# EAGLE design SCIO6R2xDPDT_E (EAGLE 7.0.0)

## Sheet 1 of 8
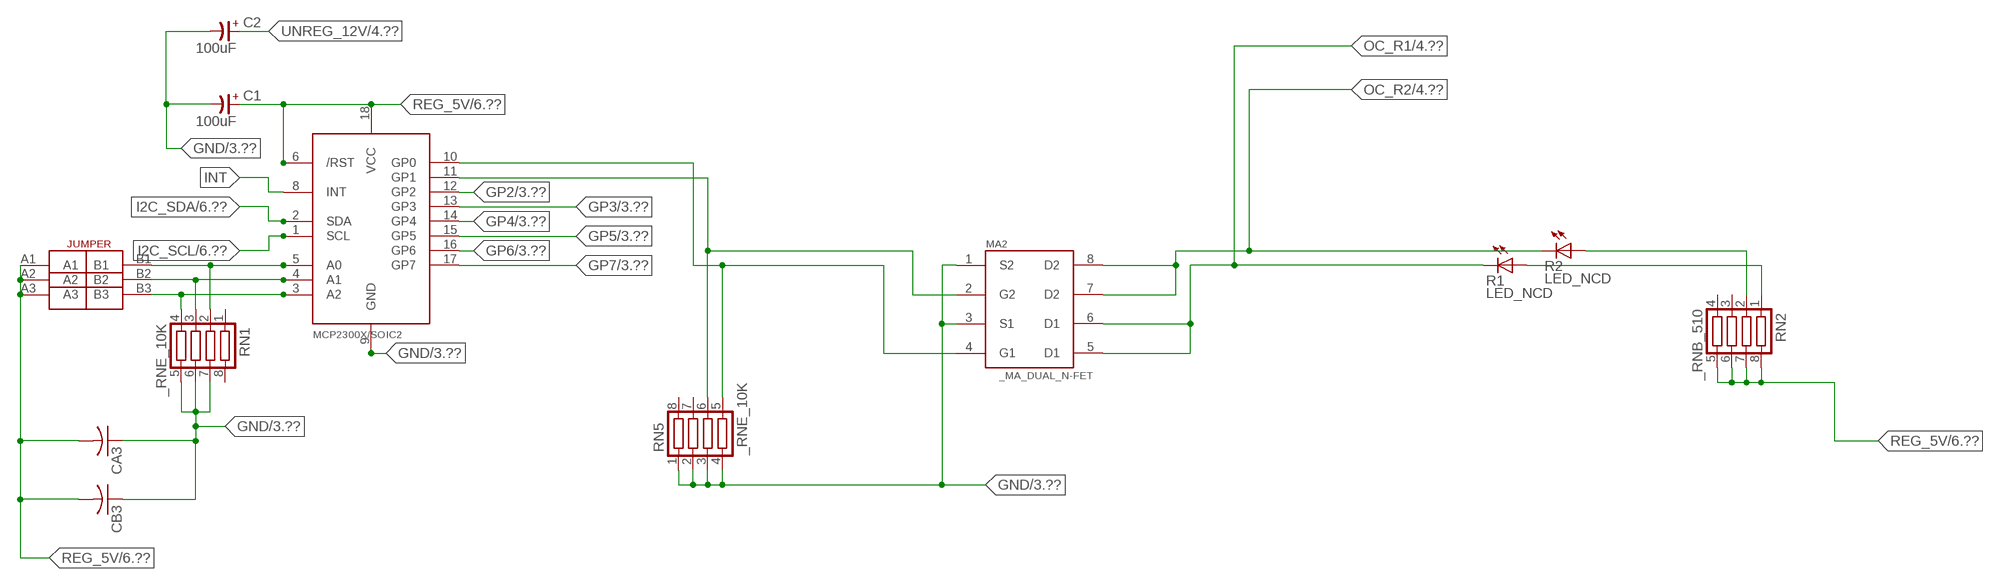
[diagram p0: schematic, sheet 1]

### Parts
C1  100uF  CP-E-025X060  [E-025X060]
C2  100uF  CP-E-025X060  [E-025X060]
CA3  CC1206KRX7R9BB104C1206K  [CC1206KRX7R9BB104]
CB3  TMK316F106ZL-TC1206K  [TMK316F106ZL-T]
IC2  MCP2300X/SO  [SO18W]
MA2  _MA_DUAL_N-FET  [_MA_DUAL_N-FET]
R1  LED_NCD  [CHIPLED_0603]
R2  LED_NCD  [CHIPLED_0603]
RN1  _RNE_10K  [RNE]
RN2  _RNB_510  [RNB]
RN5  _RNE_10K  [RNE]
U$18  JUMPER_3X2  [JUMPER_3X2]

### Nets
GND: C1.- C2.- CA3.1 CB3.1 IC2.9(GND) MA2.1(S2) MA2.3(S1) RN1.5 RN1.6 RN1.7 RN5.1 RN5.2 RN5.3 RN5.4 ; also sheet 3,6,8
GP2: IC2.12(GP2) ; also sheet 3
GP3: IC2.13(GP3) ; also sheet 3
GP4: IC2.14(GP4) ; also sheet 3
GP5: IC2.15(GP5) ; also sheet 3
GP6: IC2.16(GP6) ; also sheet 3
GP7: IC2.17(GP7) ; also sheet 3
I2C_SCL: IC2.1(SCL) ; also sheet 6
I2C_SDA: IC2.2(SDA) ; also sheet 6
INT: IC2.8(INT)
N$6: IC2.5(A0) RN1.2 U$18.B1
N$7: IC2.4(A1) RN1.3 U$18.B2
N$8: IC2.3(A2) RN1.4 U$18.B3
N$22: IC2.11(GP1) MA2.2(G2) RN5.6
N$23: IC2.10(GP0) MA2.4(G1) RN5.5
N$31: R2.A RN2.2
N$32: R1.A RN2.1
OC_R1: MA2.5(D1) MA2.6(D1) R1.C ; also sheet 4
OC_R2: MA2.7(D2) MA2.8(D2) R2.C ; also sheet 4
REG_5V: C1.+ CA3.2 CB3.2 IC2.6(/RST) IC2.18(VCC) RN2.5 RN2.6 RN2.7 RN2.8 U$18.A1 U$18.A2 U$18.A3 ; also sheet 6,8
UNREG_12V: C2.+ ; also sheet 4,6
Unconnected: RN1.1 RN1.8 RN2.3 RN2.4 RN5.7 RN5.8

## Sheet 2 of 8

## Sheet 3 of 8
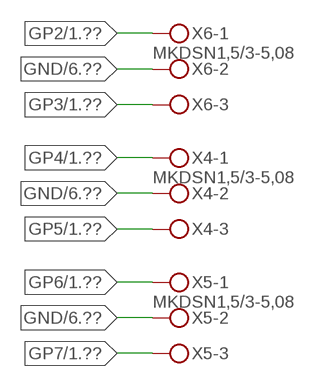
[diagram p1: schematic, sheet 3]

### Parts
X4  MKDSN1,5/3-5,08  [MKDSN1,5/3-5,08]
X5  MKDSN1,5/3-5,08  [MKDSN1,5/3-5,08]
X6  MKDSN1,5/3-5,08  [MKDSN1,5/3-5,08]

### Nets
GND: X4.2 X5.2 X6.2 ; also sheet 1,6,8
GP2: X6.1 ; also sheet 1
GP3: X6.3 ; also sheet 1
GP4: X4.1 ; also sheet 1
GP5: X4.3 ; also sheet 1
GP6: X5.1 ; also sheet 1
GP7: X5.3 ; also sheet 1

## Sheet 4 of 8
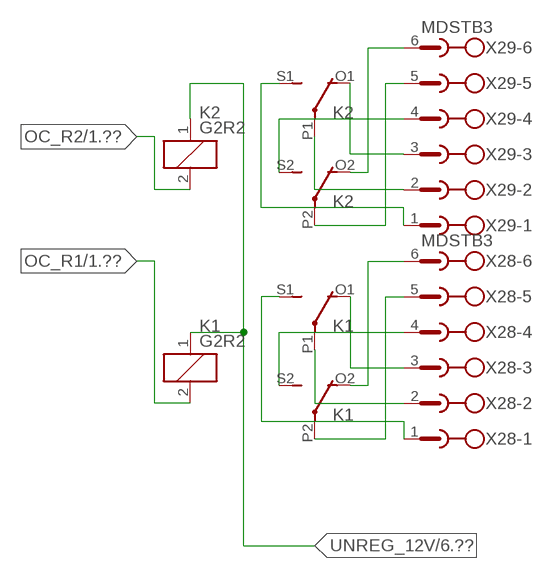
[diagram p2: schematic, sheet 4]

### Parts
K1  G2R2  [G2R2]
K2  G2R2  [G2R2]
X28  MDSTB3  [MDSTB3]
X29  MDSTB3  [MDSTB3]

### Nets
N$203: K1.P2(3:COM) X28.5
N$204: K1.O2(3:NC) X28.6
N$205: K1.S2(3:NO) X28.4
N$206: K1.P1(2:COM) X28.2
N$207: K1.O1(2:NC) X28.3
N$208: K1.S1(2:NO) X28.1
N$209: K2.P2(3:COM) X29.5
N$210: K2.O2(3:NC) X29.6
N$211: K2.S2(3:NO) X29.4
N$212: K2.S1(2:NO) X29.1
N$213: K2.P1(2:COM) X29.2
N$214: K2.O1(2:NC) X29.3
OC_R1: K1.2(1:C2) ; also sheet 1
OC_R2: K2.2(1:C2) ; also sheet 1
UNREG_12V: K1.1(1:C1) K2.1(1:C1) ; also sheet 1,6

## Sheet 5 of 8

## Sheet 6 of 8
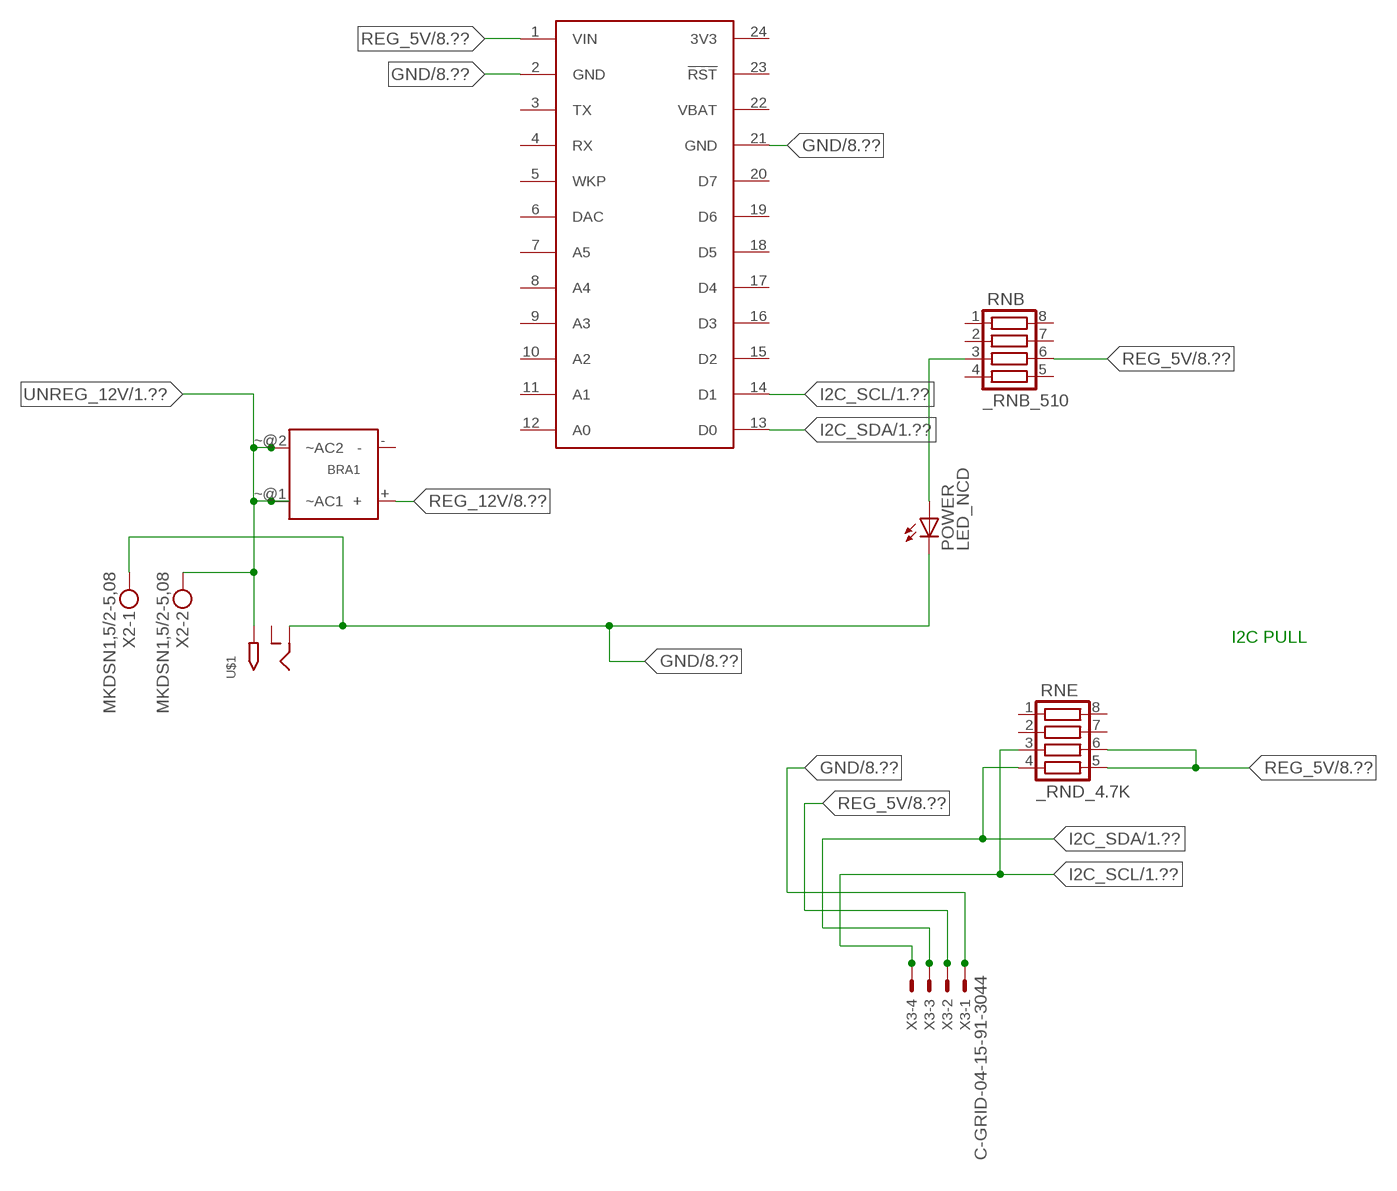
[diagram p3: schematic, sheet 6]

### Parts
BRA1  MB2S_  [MB2S]
POWER  LED_NCD  [CHIPLED_0603]
RNB  _RNB_510  [RNB]
RNE  _RND_4.7K  [RND]
S1  SPARK_CORECORE  [SPARK_CORE]
U$1  2.1MMJACK  [PJ-102A]
X2  MKDSN1,5/2-5,08  [MKDSN1,5/2-5,08]
X3  C-GRID-04-15-91-3044  [15-91-04]

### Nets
GND: POWER.C S1.2(GND) S1.21(GND) U$1.RING X2.1 X3.1 ; also sheet 1,3,8
I2C_SCL: RNE.3 S1.14(D1) X3.4 ; also sheet 1
I2C_SDA: RNE.4 S1.13(D0) X3.3 ; also sheet 1
N$2: POWER.A RNB.3
REG_5V: RNB.6 RNE.5 RNE.6 S1.1(VIN) X3.2 ; also sheet 1,8
REG_12V: BRA1.+ ; also sheet 8
UNREG_12V: BRA1.~@1(~AC1) BRA1.~@2(~AC2) U$1.TIP X2.2 ; also sheet 1,4
Unconnected: BRA1.- RNB.1 RNB.2 RNB.4 RNB.5 RNB.7 RNB.8 RNE.1 RNE.2 RNE.7 RNE.8 S1.3(TX) S1.4(RX) S1.5(WKP) S1.6(DAC) S1.7(A5) S1.8(A4) S1.9(A3) S1.10(A2) S1.11(A1) S1.12(A0) S1.15(D2) S1.16(D3) S1.17(D4) S1.18(D5) S1.19(D6) S1.20(D7) S1.23(!RST) U$1.RING_SW

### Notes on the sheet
- I2C PULL

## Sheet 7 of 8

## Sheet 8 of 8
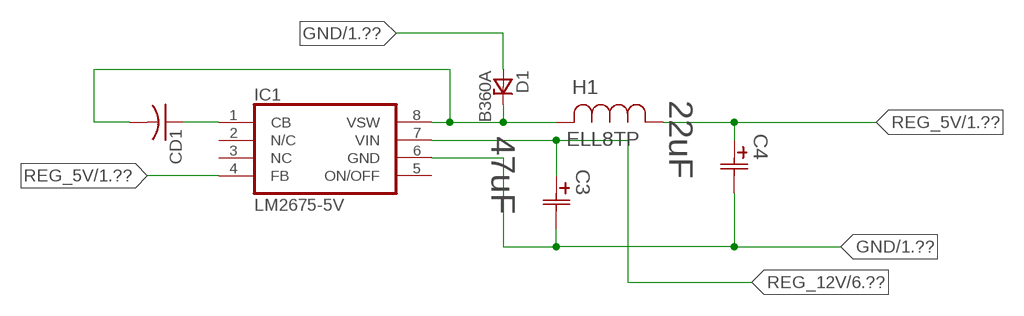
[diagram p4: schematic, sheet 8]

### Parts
C3  47uF  490-5463-6-NDCAP  [C2917(7343)-Y]
C4  22uF  490-5463-6-NDCAP  [C2917(7343)-Y]
CD1  _CD_10NF_50VC1206K  [_CD_10NF_50V]
D1  B360A  [DO214AC_ZENER]
H1  ELL8TP  [IND_ELL8TP]
IC1  LM2675-5V  LM2675  [SO-8]

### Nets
GND: C3.2(C2) C4.2(C2) D1.A IC1.6(GND) ; also sheet 1,3,6
N$1: CD1.2 D1.C H1.2 IC1.8(VSW)
N$3: CD1.1 IC1.1(CB)
REG_5V: C4.1(C1) H1.1 IC1.4(FB) ; also sheet 1,6
REG_12V: C3.1(C1) IC1.7(VIN) ; also sheet 6
Unconnected: IC1.2(N/C) IC1.5(ON/OFF)

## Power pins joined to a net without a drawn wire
3V3: S1.24(3V3)
NC: IC1.3(NC)
VBAT: S1.22(VBAT)

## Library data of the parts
BRA1 = NCD_ULTIMATE_LIBRARY:MB2S: Bridge Rectifier BRA MB2S 200V 500ma Digikey MB2S-TPMSTR-ND/MB2S-TP
C1 C2 = NCD_ULTIMATE_LIBRARY:CP-: Capacitors All Kinds POLARIZED CAP
C3 C4 = NCD_ULTIMATE_bhaskar:490-5463-6-ND: NCD CAP
CA3 = NCD_ULTIMATE_LIBRARY:CC1206KRX7R9BB104: Capacitor CA .1uF 50V SMT C1206K CC1206KRX7R9BB104
CB3 = NCD_ULTIMATE_LIBRARY:TMK316F106ZL-T: Capacitor CB 10uF SMT 1206 TMK316F106ZL-T
CD1 = NCD_ULTIMATE_LIBRARY:_CD_10NF_50V: Capacitor 10nF SMT
D1 = NCD_ULTIMATE_bhaskar:B360A: NCD DIODE B350A/B360A
H1 = NCD_ULTIMATE_bhaskar:ELL8TP: NCD coil
IC1 = NCD_ULTIMATE_bhaskar:LM2675: LM2675 NCD http://www.ti.com/lit/ds/symlink/lm2675.pdf
IC2 = NCD_ULTIMATE_LIBRARY:MCP2300X: Semiconductor Port Expander I/O 8-Bit I2C MCP23008 Inexpensive i2c i/o expander - 8 general purpose i/o pins with optional pullups
K1 K2 = NCD_ULTIMATE_LIBRARY:G2R2: RELAY 2 x switch, Omron
MA2 = NCD_ULTIMATE_LIBRARY:_MA_DUAL_N-FET: FET Dual N-Channel 8-SOIC NMOSFET Digikey 785-1064-2-ND/AO4842
POWER = NCD_ULTIMATE_bhaskar:LED_NCD
R1 R2 = NCD_ULTIMATE_LIBRARY:LED_NCD: LED Digikey 754-1132-2-ND/APT2012SRCPRV
RN1 RN5 = NCD_ULTIMATE_LIBRARY:_RNE_10K: Resistor Array RNE SMT 10K x 4 Single Resistor Source: http://www.ctscorp.com/components/Datasheets/CTSChipArrayDs.pdf Digikey 742C083103JPTR-ND/742C083103JP; OC_FARNELL: unknown; OC_NEWARK: unknown
RN2 RNB = NCD_ULTIMATE_LIBRARY:_RNB_510: Resistor Array RNB SMT 510 x 4 Single Resistor Source: http://www.ctscorp.com/components/Datasheets/CTSChipArrayDs.pdf Digikey 742C083511JPTR-ND/ 742C083511JP; OC_FARNELL: unknown; OC_NEWARK: unknown
RNE = NCD_ULTIMATE_LIBRARY:_RND_4.7K: Resistor Array RND SMT 4.7K x 4 Single Resistor Source: http://www.ctscorp.com/components/Datasheets/CTSChipArrayDs.pdf Digikey 742C083472JPTR-ND/742C083472JP; OC_FARNELL: unknown; OC_NEWARK: unknown
S1 = Spark:SPARK_CORE
U$1 = NCD_ULTIMATE_CONNECTORS:2.1MMJACK: 2.1mm x 5.5mm DC jack with internal switch. Digikey part #PJ-102A, 4UCON part #05537 By microbuilder.eu
U$18 = NCD_ULTIMATE_CONNECTORS:JUMPER_3X2
X2 = NCD_ULTIMATE_CONNECTORS:MKDSN1,5/2-5,08: MKDSN 1,5/ 2-5,08 Printklemme
X3 = NCD_ULTIMATE_CONNECTORS:C-GRID-04: CONNECTOR 4-Pos I2C wire to board 2.54 mm (0.100") pitch header Digikey WM1342-ND/0015912045; OC_FARNELL: unknown; OC_NEWARK: unknown
X4-X6 = NCD_ULTIMATE_CONNECTORS:MKDSN1,5/3-5,08: MKDSN 1,5/ 3-5,08 Printklemme Nennstrom: 13,5 A Nennspannung: 250 V Rastermaß: 5,08 mm Polzahl: 3 Anschlussart: Schraubanschluss Montage: Löten Anschlussrichtung Leiter/Platine: 0 ° Artikelnummer: 1729131 Source: http://eshop.phoenixcontact.com .. 1729131.pdf
X28 X29 = NCD_ULTIMATE_LIBRARY:MDSTB3: PHOENIX

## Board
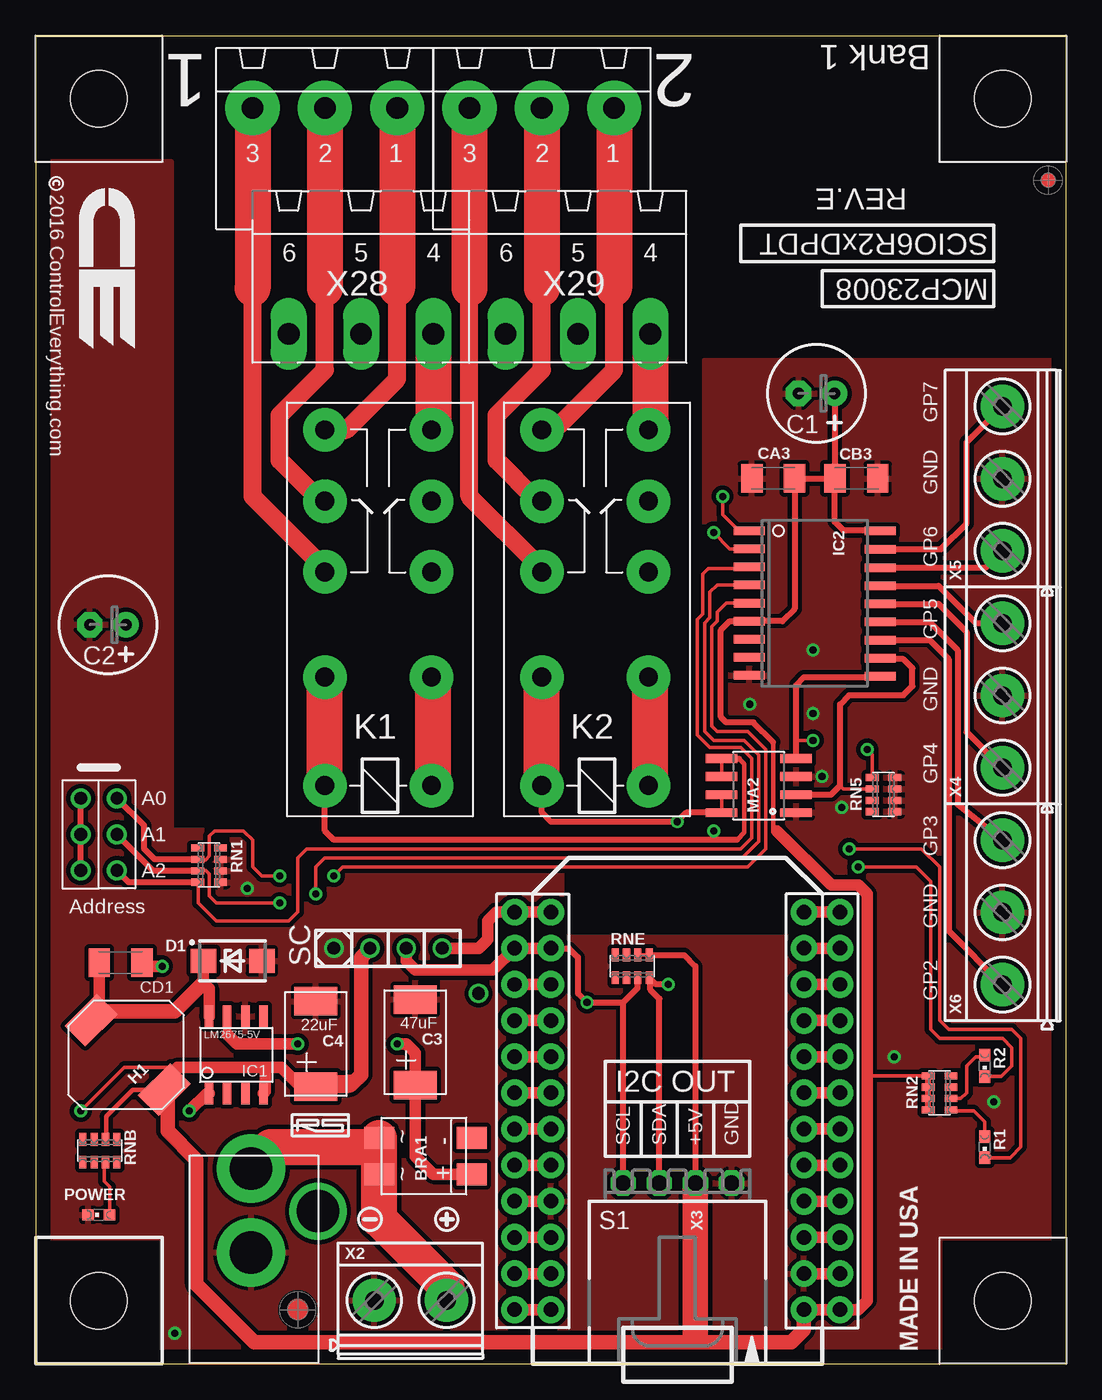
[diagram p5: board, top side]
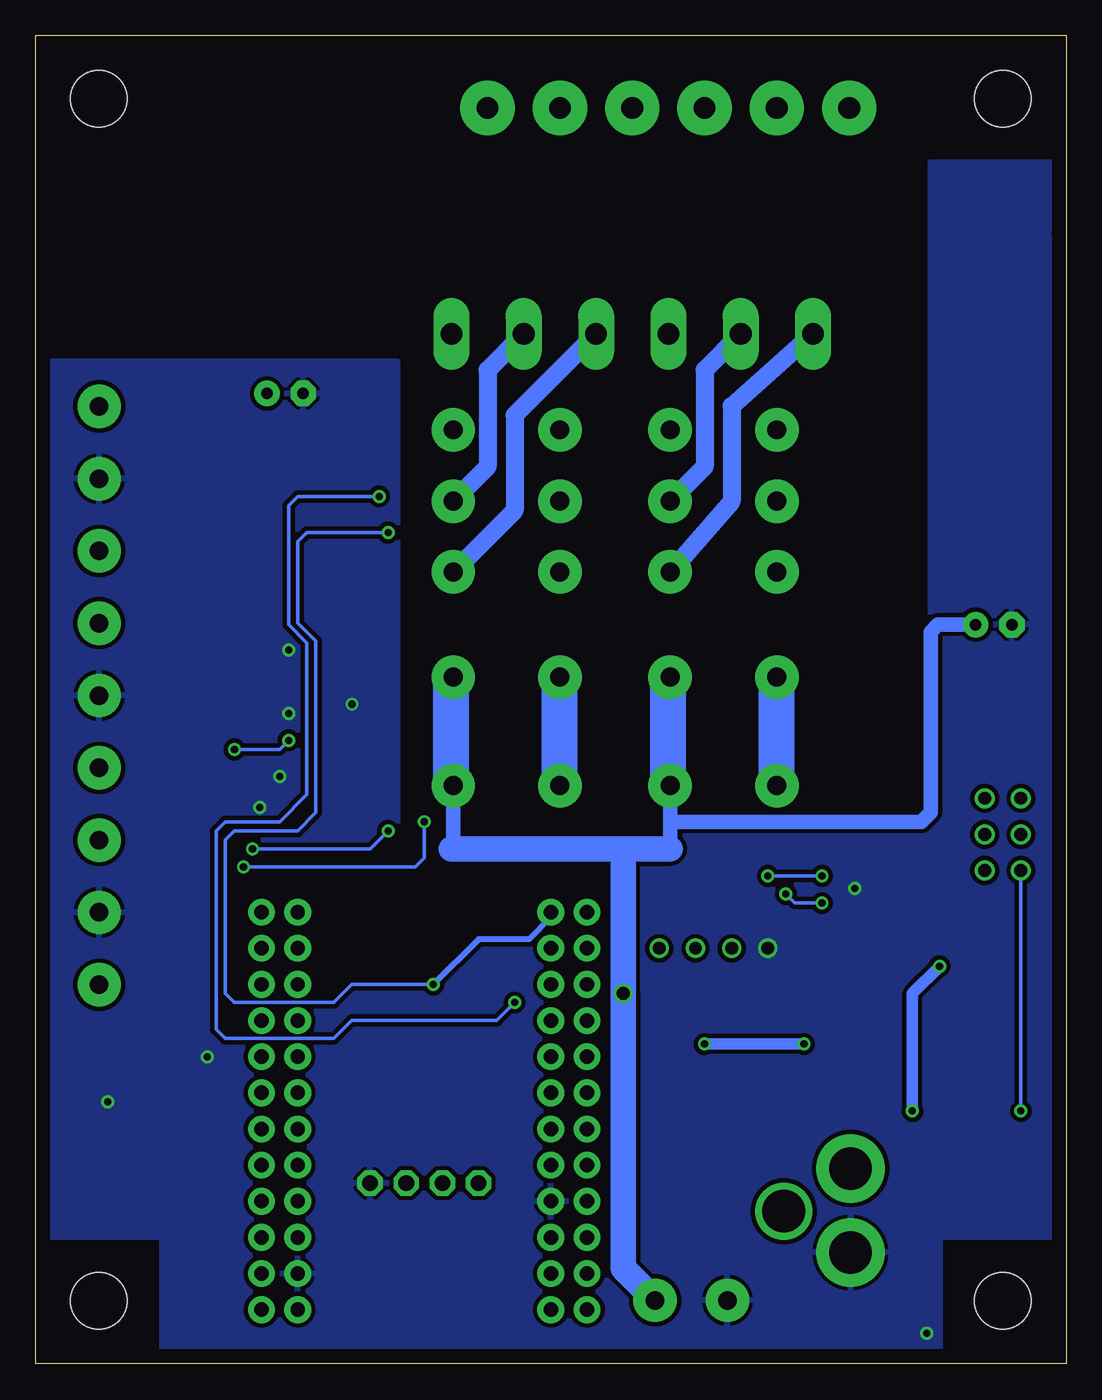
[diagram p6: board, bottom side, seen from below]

Size 72.39 x 93.34 mm. Coordinates in mm from the lower left corner, seen from the top.
Outline: 59.69,0 61.58,0
Outline: 59.69,0 72.39,0 72.39,93.34 0,93.34 0,79.38 0,0 59.69,0
Copper layers (1*16): Top 0.035mm / dielectric 1.5mm / Bottom 0.035mm
Design rules "default": minimum track width 10mil, minimum drill 24mil, track to track 8mil, track to pad 8mil, pad to pad 8mil, via to via 8mil, smd to smd 8mil, copper to edge 40mil, drill to drill 8mil, minimum pad ring 10mil, minimum via ring 8mil, stop-mask expansion 4mil, vias tented up to drill 0mil, thermal gap 10mil
Holes 3.96 mm at 4.45,4.45 4.45,4.45

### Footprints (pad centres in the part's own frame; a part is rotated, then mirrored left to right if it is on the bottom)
MB2S = smd 1.55 x 2.1: + 0,-6.5; - 2.54,-6.5; ~@1 0,0; ~@2 2.54,0
E-025X060 = drill 0.813 pad 1.778: + -1.27,0 | drill 0.813 pad 1.778 octagon: - 1.27,0
C2917(7343)-Y = smd 2 x 3: 1 -3,0; 2 3,0
CC1206KRX7R9BB104 = smd 1.5 x 2: 1 -1.5,0; 2 1.5,0
TMK316F106ZL-T = smd 1.5 x 2: 1 -1.5,0; 2 1.5,0
_CD_10NF_50V = smd 1.5 x 2: 1 -1.5,0; 2 1.5,0
DO214AC_ZENER = smd 1.8 x 1.7: A 2.05,0; C -2.05,0
IND_ELL8TP = smd 2.054 x 3.2 rotated 45: 1 -2.442,-2.696; 2 2.442,2.442
SO-8 = smd 0.6 x 1.55: 1 -1.905,-2.69; 2 -0.635,-2.69; 3 0.635,-2.69; 4 1.905,-2.69; 5 1.905,2.71; 6 0.635,2.71; 7 -0.635,2.71; 8 -1.905,2.71
SO18W = smd 0.6 x 2.2: 1 -4.445,-4.6; 2 -3.175,-4.6; 3 -1.905,-4.6; 4 -0.635,-4.6; 5 0.635,-4.6; 6 1.905,-4.6; 7 3.175,-4.6; 8 4.445,-4.6; 9 5.715,-4.6; 10 5.775,4.6; 11 4.505,4.6; 12 3.235,4.6; 13 1.965,4.6; 14 0.695,4.6; 15 -0.575,4.6; 16 -1.845,4.6; 17 -3.145,4.6; 18 -4.445,4.6
G2R2 = drill 1.321 pad 3.048: 1 -2.54,-3.683; 2 -2.54,3.81; 3 5.08,-3.683; 4 5.08,3.81; O1 12.471,3.81; O2 12.471,-3.683; P1 17.45,3.81; P2 17.45,-3.683; S1 22.454,3.81; S2 22.454,-3.683
_MA_DUAL_N-FET = smd 0.61 x 2.21: 1 -1.905,-2.616; 2 -0.635,-2.616; 3 0.635,-2.616; 4 1.905,-2.616; 5 1.905,2.616; 6 0.635,2.616; 7 -0.635,2.616; 8 -1.905,2.616
CHIPLED_0603 = smd 0.8 x 0.8: A 0,-0.75; C 0,0.75
CHIPLED_0603' = smd 0.8 x 0.876: A 0,-0.75; C 0,0.75
RNE = smd 0.5 x 0.9: 1 -1.2,-0.8; 2 -0.4,-0.8; 3 0.4,-0.8; 4 1.2,-0.8; 5 1.2,0.8; 6 0.4,0.8; 7 -0.4,0.8; 8 -1.2,0.8
RNB = smd 0.5 x 0.9: 1 -1.2,-0.8; 2 -0.4,-0.8; 3 0.4,-0.8; 4 1.2,-0.8; 5 1.2,0.8; 6 0.4,0.8; 7 -0.4,0.8; 8 -1.2,0.8
RND = smd 0.5 x 0.9: 1 -1.2,-0.8; 2 -0.4,-0.8; 3 0.4,-0.8; 4 1.2,-0.8; 5 1.2,0.8; 6 0.4,0.8; 7 -0.4,0.8; 8 -1.2,0.8
SPARK_CORE = drill 1.016 pad 1.88: 1 -8.89,13.97; 2 -8.89,11.43; 3 -8.89,8.89; 4 -8.89,6.35; 5 -8.89,3.81; 6 -8.89,1.27; 7 -8.89,-1.27; 8 -8.89,-3.81; 9 -8.89,-6.35; 10 -8.89,-8.89; 11 -8.89,-11.43; 12 -8.89,-13.97; 13 8.89,-13.97; 14 8.89,-11.43; 15 8.89,-8.89; 16 8.89,-6.35; 17 8.89,-3.81; 18 8.89,-1.27; 19 8.89,1.27; 20 8.89,3.81; 21 8.89,6.35; 22 8.89,8.89; 23 8.89,11.43; 24 8.89,13.97; 25 -11.43,13.97; 26 -11.43,11.43; 27 -11.43,8.89; 28 -11.43,6.35; 29 -11.43,3.81; 30 -11.43,1.27; 31 -11.43,-1.27; 32 -11.43,-3.81; 33 -11.43,-6.35; 34 -11.43,-8.89; 35 -11.43,-11.43; 36 -11.43,-13.97; 37 11.43,13.97; 38 11.43,11.43; 39 11.43,8.89; 40 11.43,6.35; 41 11.43,3.81; 42 11.43,1.27; 43 11.43,-1.27; 44 11.43,-3.81; 45 11.43,-6.35; 46 11.43,-8.89; 47 11.43,-11.43; 48 11.43,-13.97
PJ-102A = drill 3 pad 4.8: RING 0.1,-3.39; TIP 0.1,-9.29 | drill 3 pad 3.251: RING_SW -4.6,-6.29
PCB_MOUNTING_HOLE = hole 3.962: 4.445,4.445
JUMPER_3X2 = drill 0.9: A1 0,5.08; A2 0,2.54; A3 0,0; B1 2.54,5.08; B2 2.54,2.54; B3 2.54,0
MKDSN1,5/2-5,08 = drill 1.3 pad 3.048: 1 -2.561,0.025; 2 2.519,0.025
15-91-04 = drill 1.1 pad 1.778 octagon: 1 -3.81,-7.62; 2 -1.27,-7.62; 3 1.27,-7.62; 4 3.81,-7.62
MKDSN1,5/3-5,08 = drill 1.3 pad 3.048: 1 -7.641,0.025; 2 -2.561,0.025; 3 2.519,0.025
MDSTB3 = drill 1.524 pad 3.81: 1 -3.81,-10.795; 2 1.27,-10.795; 3 6.35,-10.795 | drill 1.524 pad 2.54 long: 4 -6.35,5.08; 5 -1.27,5.08; 6 3.81,5.08

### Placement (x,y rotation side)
BRA1  24.13,13.34 90 top
C1  54.86,68.2 180 top
C2  5.08,51.94 180 top
C3  26.67,22.61 90 top
C4  19.68,22.48 90 top
CA3  51.82,62.23 0 top
CB3  57.66,62.23 180 top
CD1  5.97,28.19 180 top
D1  13.84,28.32 0 top
H1  6.35,21.72 90 top
IC1  14.1,21.72 0 top
IC2  54.74,54.1 270 top
K1  24.13,43.18 90 top
K2  39.37,43.18 90 top
MA2  50.8,40.64 90 top
POWER  4.45,10.48 90 top
R1  LED_NCD  [CHIPLED_0603']  66.67,15.24 180 top
R2  LED_NCD  [CHIPLED_0603']  66.67,20.96 180 top
RN1  12.19,35.05 270 top
RN2  63.5,19.05 90 top
RN5  59.56,40 90 top
RNB  4.51,14.99 0 top
RNE  41.91,27.94 0 top
S1  45.09,17.78 180 top
U$1  15.24,4.45 180 top
U$4  PCB_MOUNTING_HOLE  [PCB_MOUNTING_HOLE]  72.39,84.45 90 top
U$6  PCB_MOUNTING_HOLE  [PCB_MOUNTING_HOLE]  72.39,0 90 top
U$7  PCB_MOUNTING_HOLE  [PCB_MOUNTING_HOLE]  8.89,84.45 90 top
U$10  [VISION_REF15]  18.41,3.81 0 top
U$18  3.17,34.67 0 top
U$19  [VISION_REF10]  71.12,83.19 0 top
U$21  [ICON_USA]  61.98,0.89 90 top
U$22  [ICON_MINUS]  23.5,10.16 180 top
U$24  [ICON_PLUS]  28.89,10.16 90 top
X2  26.35,4.45 0 top
X3  45.09,5.08 180 top
X4  67.94,49.53 90 top
X5  67.94,64.77 90 top
X6  67.94,34.29 90 top
X28  21.59,77.47 180 top
X29  36.83,77.47 180 top

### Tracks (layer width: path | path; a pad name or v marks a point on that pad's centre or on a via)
GND  (via drill 0.5, 0.9)
  other vias: 14.86,33.4 54.61,45.72 54.61,50.16 67.31,18.41 50.16,46.35 55.24,41.27 9.78,2.16 20.95,29.21 60.33,21.59 56.64,39.12
  pour Bottom (isolate 0.305): -2.54,8.89 8.89,8.89 8.89,0 63.5,0 63.5,8.89 71.75,8.89 71.75,70.48 46.99,70.48 46.99,37.46 9.53,37.46 9.53,84.45 -2.54,84.45
  pour Top (isolate 0.305): -5.08,8.89 8.89,8.89 8.89,0 63.5,0 63.5,8.89 71.75,8.89 71.75,70.48 46.99,70.48 46.99,37.46 9.53,37.46 9.53,84.45 -5.08,84.45
GP2
  Top 0.406: IC2.12 62.8,50.87 64.14,49.53 64.14,30.43 X6.1
GP3
  Top 0.406: IC2.13 62.8,52.14 64.77,50.16 64.77,39.32 X6.3
GP4
  Top 0.406: IC2.14 63.43,53.41 65.41,51.43 65.41,44.4 X4.1
GP5
  Top 0.406: IC2.15 63.43,54.68 66.04,52.07 67.9,52.07 X4.3
GP6
  Top 0.406: IC2.16 66.74,55.95 X5.1
GP7
  Top 0.406: IC2.17 63.6,57.25 65.41,59.05 65.41,64.77 X5.3
I2C_SCL  (via drill 0.5, 0.9)
  Top 0.254: IC2.1 49.4,58.55 48.26,59.69 v48.26,60.96
  Top 0.406: X3.4 41.27,25.4 | 41.27,25.4 42.29,26.42 42.29,27.12 RNE.3 | S1.14 37.47,29.21 38.1,28.57 38.1,26.04 v38.73,25.4 41.27,25.4
  Top 0.813: v26.04,29.21 26.04,28.32 26.67,27.69 32.13,27.69 33.66,29.21
  Bottom 0.254: v48.26,60.96 53.98,60.96 54.61,60.32 54.61,51.94 53.34,50.67 53.34,40 55.24,38.1 59.05,38.1 59.69,37.46 59.69,23.5 59.05,22.86 51.44,22.86 50.16,24.13 40.01,24.13 v38.73,25.4
I2C_SDA  (via drill 0.5, 0.9)
  Top 0.254: IC2.2 48.77,57.28 v47.62,58.42
  Top 0.406: X3.3 43.81,25.65 43.18,26.29 43.18,27.07 RNE.4 43.58,26.67 v44.45,26.67
  Top 0.813: v28.57,29.21 31.11,29.21 31.75,29.85 31.75,31.12 32.38,31.75 33.66,31.75
  Bottom 0.254: v47.62,58.42 53.34,58.42 53.98,57.78 53.98,52.07 52.7,50.8 52.7,38.73 53.98,37.46 58.42,37.46 59.05,36.83 59.05,26.04 58.42,25.4 51.44,25.4 50.16,26.67 v44.45,26.67
  Bottom 0.406: S1.13 36.2,31.37 37.72,29.85 41.27,29.85 v44.45,26.67
N$1
  Top 0.813: H1.2 3.88,24.77 | D1.C 11.79,26.78 12.19,26.38 IC1.8 | CD1.2 4.47,24.79 4.45,24.77
  Top 1.016: 3.88,24.77 4.45,24.77 9.78,24.77 11.79,26.78
N$2
  Top 0.254: POWER.A 5.2,12.46 4.83,12.83 4.83,14.1 RNB.3
  Top 0.406: 4.95,14.14 RNB.3
N$3  (via drill 0.5)
  Top 0.813: IC1.1 12.04,19.03 v10.79,17.78 | v8.89,27.94 7.72,27.94 CD1.1
  Bottom 0.813: v10.79,17.78 10.79,26.04 v8.89,27.94
N$6  (via drill 0.5)
  Top 0.254: v20.95,34.29 21.59,34.92 50.04,34.92 51.31,36.2 51.31,43.18 50.04,44.45 47.88,44.45 47.5,44.83 47.5,51.82 47.88,52.2 47.88,52.83 48.51,53.47 IC2.5 50.01,53.34 | v17.14,34.29 15.88,34.29 15.24,34.92 15.24,36.83 14.61,37.46 12.57,37.46 12.19,37.08 12.19,35.69 11.94,35.43 11.41,35.43 RN1.2
  Top 0.406: RN1.2 8.36,35.45 7.62,36.2 7.62,37.85 U$18.B1
  Bottom 0.254: v20.95,34.29 v17.14,34.29
N$7  (via drill 0.5)
  Top 0.254: v19.68,33.02 19.68,34.92 20.32,35.56 49.66,35.56 50.8,36.7 50.8,42.8 49.78,43.81 47.62,43.81 46.99,44.45 46.99,52.07 47.37,52.45 47.37,54.23 47.88,54.74 IC2.4 50.01,54.61 | v17.14,32.38 12.7,32.38 12.19,32.89 12.19,34.42 11.94,34.67 11.41,34.67 RN1.3
  Top 0.406: RN1.3 8.27,34.65 U$18.B2
  Bottom 0.254: v19.68,33.02 19.05,32.38 v17.14,32.38
N$8
  Top 0.254: RN1.4 11.43,33.81 11.43,32.38 12.7,31.12 17.78,31.12 18.41,31.75 18.41,35.56 19.05,36.2 49.53,36.2 50.29,36.96 50.29,42.54 49.53,43.31 47.37,43.31 46.48,44.2 46.48,52.32 46.86,52.7 46.86,55.5 47.24,55.88 50.01,55.88 IC2.3
  Top 0.406: RN1.4 6.53,33.85 U$18.B3
N$22
  Top 0.254: RN5.6 56.75,40.4 56.52,40.64
  Top 0.406: MA2.2 55.88,40 56.52,40.64 56.52,46.35 57.15,46.99 60.96,46.99 61.59,47.62 61.59,48.89 60.96,49.53 59.4,49.53 IC2.11
N$23  (via drill 0.5)
  Top 0.254: RN5.5 58.76,42.84 v58.42,43.18 | v54.61,43.81 53.42,43.81
  Top 0.406: MA2.4 53.42,43.81 53.42,47.7 53.98,48.26 59.27,48.26 IC2.10
  Bottom 0.254: v58.42,43.18 55.24,43.18 v54.61,43.81
N$31
  Top 0.254: RN2.2 65,18.65 65.41,19.05 65.41,20.96 66.04,21.59 66.56,21.59 R2.A
N$32
  Top 0.254: R1.A 66.67,17.02 65.91,17.78 64.37,17.78 RN2.1
N$203
  Bottom 1.27: X28.5 25.4,69.85 25.4,63.04 K1.P2
N$204
  Bottom 1.27: X28.6 23.5,67.31 23.5,60.6 K1.O2
N$205
  Top 2.54: X28.4 27.94,65.76 K1.S2
N$206
  Top 1.27: K1.P1 20.02,60.63 17.14,63.5 17.14,66.67 20.32,69.85 20.32,75.56
  Top 2.54: X28.2 20.32,75.56
N$207
  Top 1.27: K1.O1 20.32,55.88 15.24,60.96 15.24,75.56
  Top 2.54: X28.3 15.24,75.56
N$208
  Top 1.27: 25.4,75.56 25.4,69.22 21.82,65.63 K1.S1
  Top 2.54: X28.1 25.4,75.56
N$209
  Bottom 1.27: X29.5 40.64,69.85 40.64,63.04 K2.P2
N$210
  Bottom 1.27: X29.6 38.73,66.67 38.73,59.97 K2.O2
N$211
  Top 2.54: X29.4 43.18,65.76 K2.S2
N$212
  Top 1.27: 40.64,75.56 40.64,69.85 36.42,65.63 K2.S1
  Top 2.54: X29.1 40.64,75.56
N$213
  Top 1.27: K2.P1 35.26,60.63 32.38,63.5 32.38,66.67 35.56,69.85 35.56,75.56
  Top 2.54: X29.2 35.56,75.56
N$214
  Top 1.27: K2.O1 35.56,55.88 30.48,60.96 30.48,75.56
  Top 2.54: X29.3 30.48,75.56
OC_R1  (via drill 0.5)
  Top 0.254: MA2.5 MA2.6 | R1.C 68.47,14.49 69.22,15.24 69.22,22.86 68.58,23.5 64.14,23.5 63.5,24.13 63.5,34.92 62.23,36.2 v57.15,36.2 | v47.62,37.46 47.62,36.83
  Top 0.305: 49.4,42.54 49.78,42.16 49.78,37.34 49.28,36.83
  Top 0.406: MA2.5 49.4,42.54 | 49.28,36.83 47.62,36.83 20.95,36.83 20.32,37.46 K1.2
  Bottom 0.254: v57.15,36.2 48.9,36.2 v47.62,37.46
OC_R2  (via drill 0.5)
  Top 0.254: MA2.7 MA2.8 | R2.C 67.83,20.21 68.58,20.96 68.58,22.23 67.94,22.86 63.5,22.86 62.87,23.5 62.87,33.91 61.85,34.92 v57.78,34.92
  Top 0.406: MA2.8 45.72,38.73 v45.09,38.1 36.2,38.1 35.56,38.73 K2.2
  Bottom 0.254: v57.78,34.92 45.72,34.92 45.09,35.56 v45.09,38.1
REG_5V  (via drill 0.5, 0.9)
  Top 0.254: RNE.6 RNE.5 | RN2.5 58.49,20.25 58.42,20.32 | 9.96,20.83 6.22,20.83 v3.17,17.78 | 51.82,37.46 52.07,37.46
  Top 0.305: 51.82,37.46 51.82,43.69 | H1.1 6.83,19.28 4.95,17.4 4.95,15.83 RNB.6
  Top 0.406: U$18.A3 U$18.A2 U$18.A1 | RN2.8 RN2.7 RN2.6 RN2.5 | 51.82,43.69 50.42,45.08 48.51,45.08 48.13,45.47 48.13,51.56 48.77,52.2 IC2.6 52.45,52.2 53.32,53.06 CA3.2 CB3.2 56.13,62.21 | IC2.18 56.77,58.55 56.13,59.18 56.13,62.21 | C1.+ 56.13,62.21 | RNE.5 45.55,28.74 46.35,27.94 X3.2
  Top 0.813: 16.13,20.83 9.96,20.83 H1.1 | 16.13,20.83 17.27,20.83 18.41,19.69 20.75,19.69 C4.1 | IC1.4 16.13,19.15 16.13,20.83 | S1.1 57.78,3.81 58.42,4.45 58.42,20.32 58.42,33.02 57.78,33.66 55.88,33.66 52.07,37.46
  Top 1.016: 46.35,2.16 46.35,1.52 | 46.35,1.52 15.37,1.52 11.3,5.59 11.3,14.35 9.27,16.38 9.27,18.41 H1.1 | 22.05,19.69 22.23,19.69 22.86,20.32 22.86,28.57 v23.5,29.21 | S1.1 53.98,2.41 53.09,1.52 46.35,1.52
  Top 1.27: 20.75,19.69 22.05,19.69
  Top 1.778: X3.2 46.35,2.16
  Bottom 0.254: v3.17,17.78 U$18.A3
REG_12V  (via drill 0.5)
  Top 0.61: IC1.7 13.46,23.16 | 14.1,22.48 14.15,22.48
  Top 0.813: v18.41,22.48 14.15,22.48 13.46,23.16 | v25.4,22.48 26.04,22.48 26.67,21.84 C3.1 26.67,14.61 27.94,13.34 BRA1.+
  Bottom 0.813: v18.41,22.48 v25.4,22.48
UNREG_12V  (via drill 0.9)
  Top 2.54: X2.2 28.87,5.42 24.13,10.16 BRA1.~@1 24.13,15.24 | 24.13,15.24 BRA1.~@2 | U$1.TIP 15.14,13.87 16.51,15.24 24.13,15.24
  Bottom 0.406: 27.81,36.2 27.81,35.69 28.57,36.2
  Bottom 1.016: K1.1 27.81,38.1 | 27.81,38.1 27.81,36.32 27.94,36.2 | K2.1 43.05,36.32 43.18,36.2 | C2.+ 9.02,51.94 9.53,51.43 9.53,38.73 10.16,38.1 27.81,38.1
  Bottom 1.778: 43.18,36.2 31.11,36.2 | 31.11,36.2 28.57,36.2 27.94,36.2 27.81,36.2 | X2.2 31.11,6.71 v31.11,26.04 31.11,36.2

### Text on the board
tNames: Bank 1 | 1 | 2 | 2016 ControlEverything.com | REV.E | SCIO6R2xDPDT | MCP23008 | GP7 | GND | GP6 | GP5 | GND | GP4 | A0 | A1 | GP3 | A2 | Address | GND | SC | GP2 | I2C OUT | SCL | SDA | +5V | GND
